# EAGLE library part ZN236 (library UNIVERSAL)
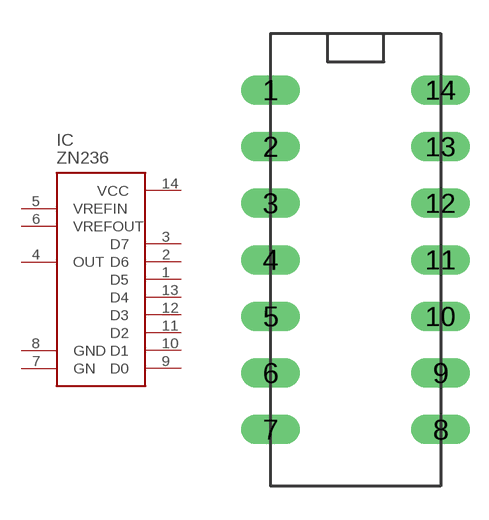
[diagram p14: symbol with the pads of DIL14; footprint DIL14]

Designator prefix IC

## ZN236  [DIL14]
1  D5  in
2  D6  in
3  D7  in
4  OUT  out
5  VREFIN  in
6  VREFOUT  sup
7  GN  sup
8  GND  sup
9  D0  in
10  D1  in
11  D2  in
12  D3  in
13  D4  in
14  VCC  sup

## Footprint DIL14 (pad centres in mm)
drill 0.813 pad 1.092 long: 1 0,0; 2 0,-2.54; 3 0,-5.08; 4 0,-7.62; 5 0,-10.16; 6 0,-12.7; 7 0,-15.24; 8 7.62,-15.24; 9 7.62,-12.7; 10 7.62,-10.16; 11 7.62,-7.62; 12 7.62,-5.08; 13 7.62,-2.54; 14 7.62,0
